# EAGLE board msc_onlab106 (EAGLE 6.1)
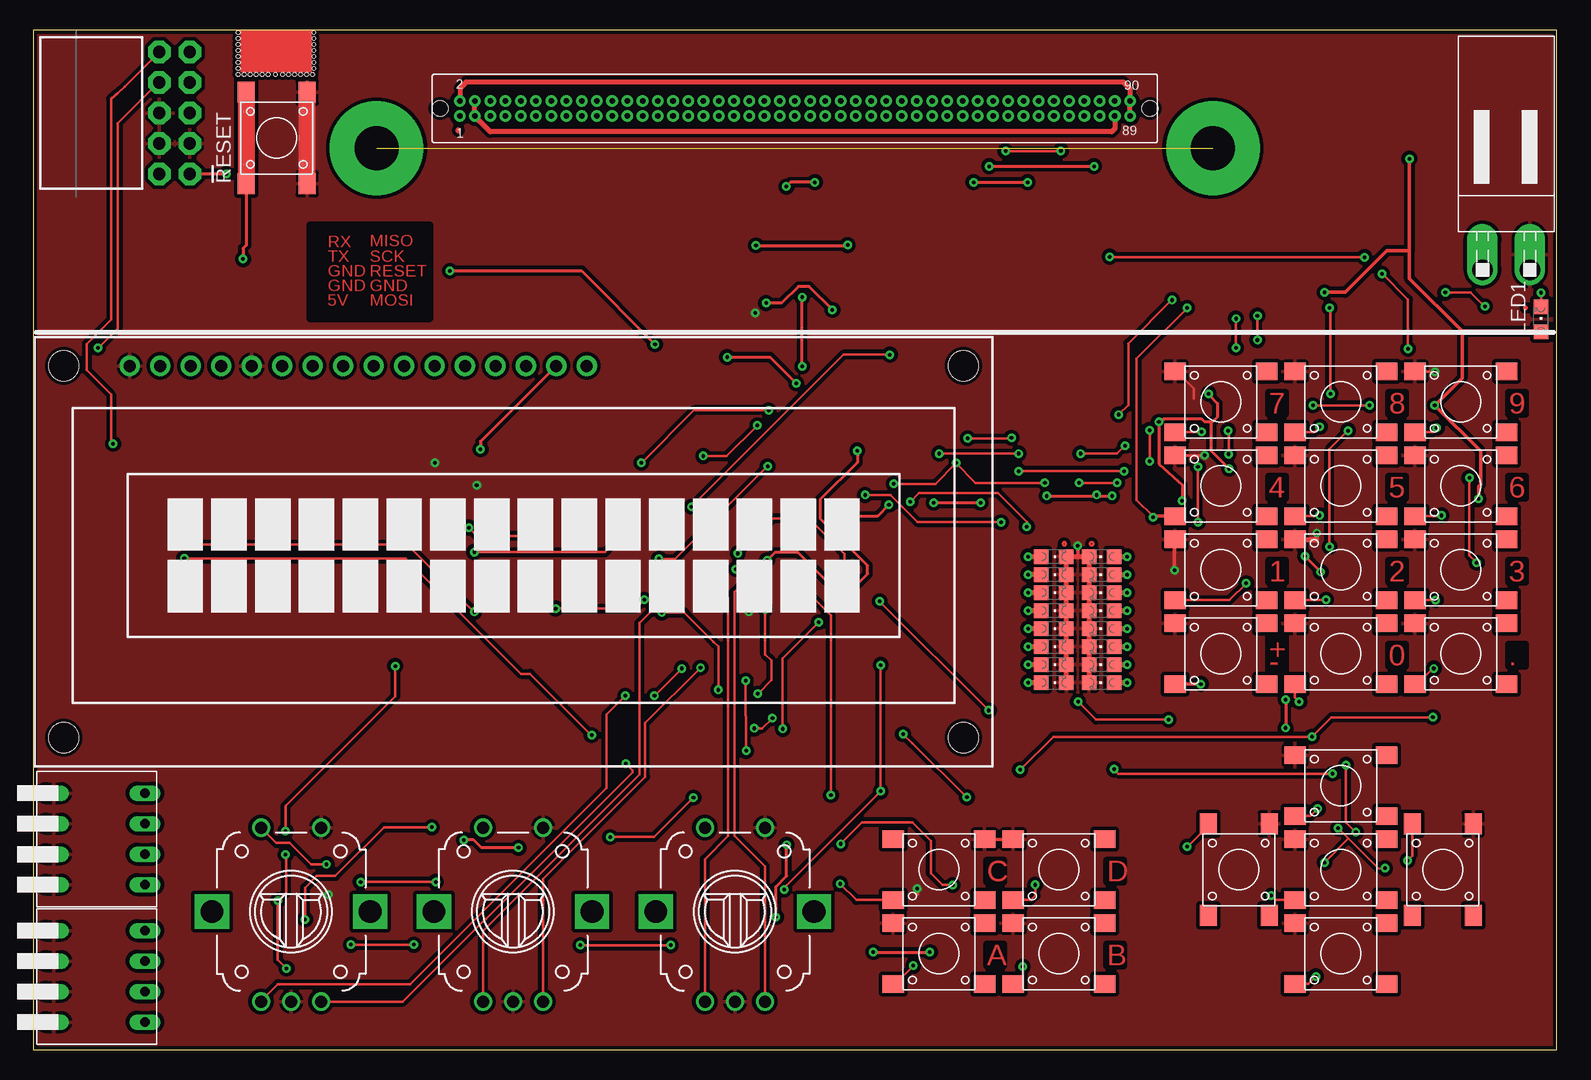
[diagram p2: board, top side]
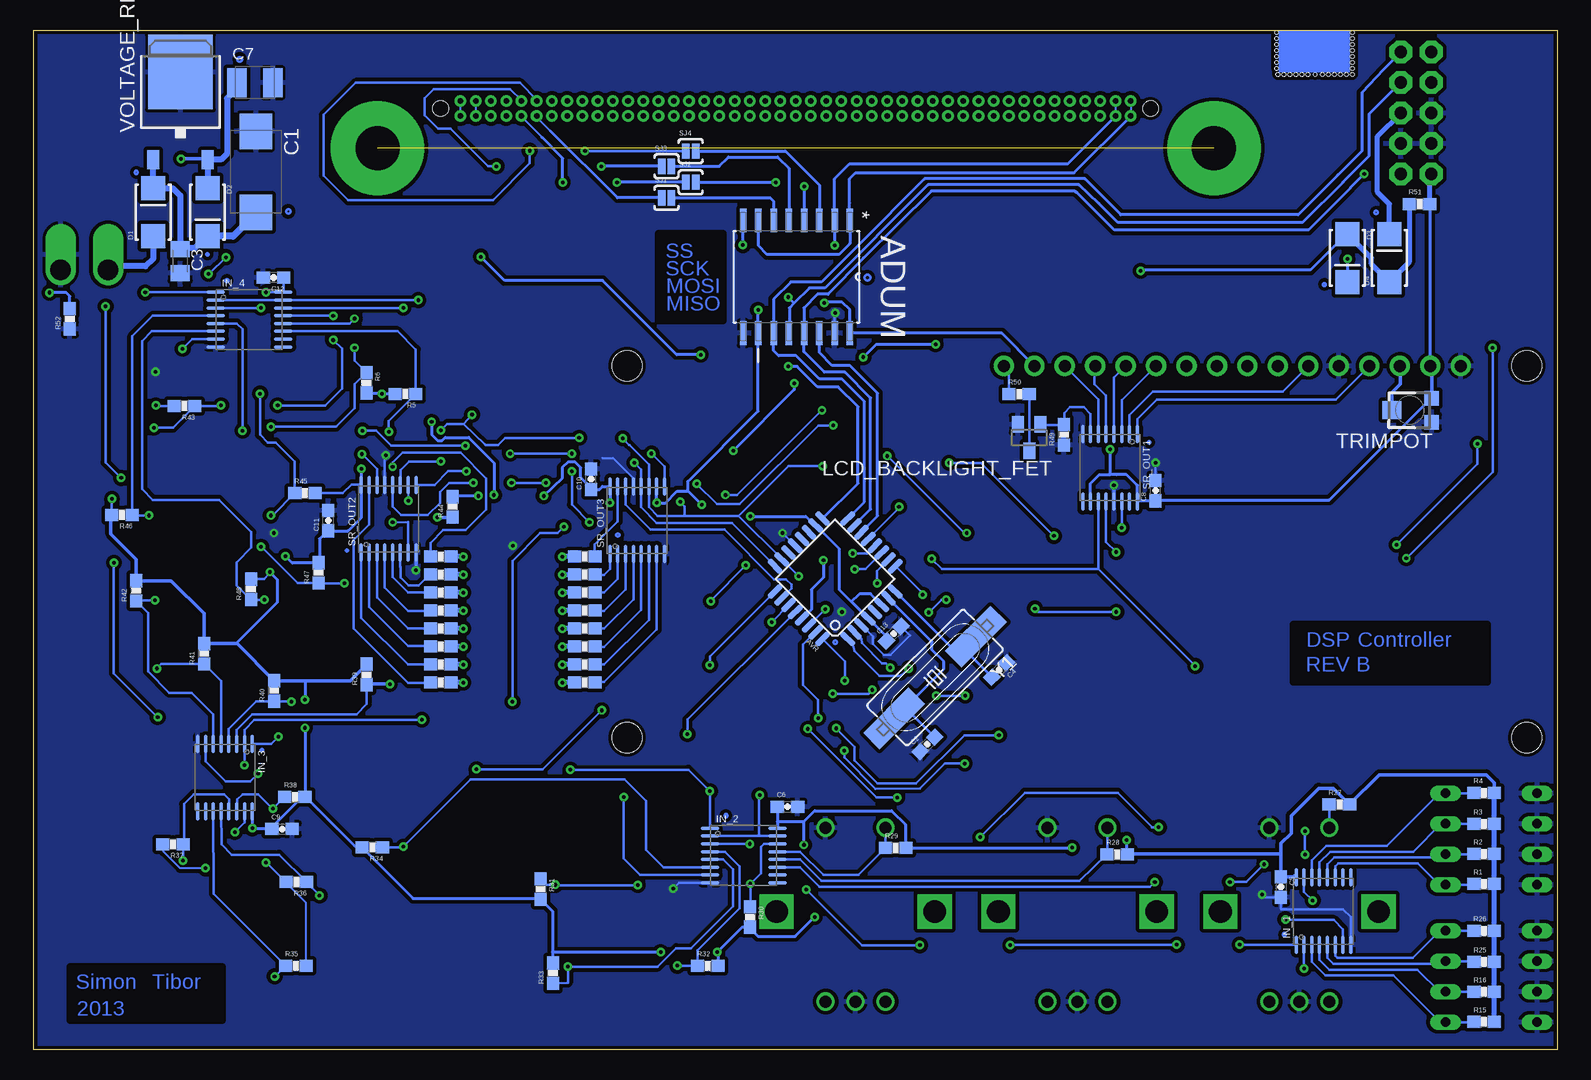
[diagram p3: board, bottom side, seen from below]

Size 127 x 85 mm. Coordinates in mm from the lower left corner, seen from the top.
Outline: 0,0 127,0 127,85 0,85 0,0
Copper layers (1*16): Top 0.035mm / dielectric 1.5mm / Bottom 0.035mm
Design rules: minimum track width 7mil, minimum drill 0.3mm, track to track 8mil, track to pad 8mil, pad to pad 7mil, via to via 7mil, smd to smd 7mil, copper to edge 10mil, drill to drill 7mil, minimum pad ring 10mil, minimum via ring 8mil, stop-mask expansion 2mil, vias tented up to drill 30mil, thermal gap 10mil
Holes 0.3 mm at 17.1,84.8 17.1,84.3 17.1,83.8 17.1,83.3 17.1,82.8 17.1,82.3 17.1,81.8 17.1,81.3 17.6,81.3 18.1,81.3 18.6,81.3 19.1,81.3 19.6,81.3 20.2,81.3 20.8,81.3 21.3,81.3 21.8,81.3 22.3,81.3 22.8,81.3 23.3,81.3 23.4,81.8 23.4,82.3 23.4,82.8 23.4,83.3 23.4,83.8 23.4,84.3 23.4,84.8
tRestrict: area 23.1,60.9 to 33.1,68.7
bRestrict: area 5.8,30.6 to 22,35.4; area 111.3,2.4 to 124,6.9; area 69.5,60.8 to 74.9,68

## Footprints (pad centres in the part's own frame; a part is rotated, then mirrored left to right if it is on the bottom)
SMD = smd 1.778 x 1.422: P$1 3.81,-2.54; P$2 -3.81,-2.54; P$3 3.81,2.54; P$4 -3.81,2.54
SOIC127P1032X265-16N = smd 1.981 x 0.533: 1 -4.699,4.445; 2 -4.699,3.175; 3 -4.699,1.905; 4 -4.699,0.635; 5 -4.699,-0.635; 6 -4.699,-1.905; 7 -4.699,-3.175; 8 -4.699,-4.445; 9 4.699,-4.445; 10 4.699,-3.175; 11 4.699,-1.905; 12 4.699,-0.635; 13 4.699,0.635; 14 4.699,1.905; 15 4.699,3.175; 16 4.699,4.445
TQFP32-08 = smd 1.524 x 0.559: 1 -4.293,2.8; 2 -4.293,2; 3 -4.293,1.2; 4 -4.293,0.4; 5 -4.293,-0.4; 6 -4.293,-1.2; 7 -4.293,-2; 8 -4.293,-2.8; 17 4.293,-2.8; 18 4.293,-2; 19 4.293,-1.2; 20 4.293,-0.4; 21 4.293,0.4; 22 4.293,1.2; 23 4.293,2; 24 4.293,2.8 | smd 0.559 x 1.524: 9 -2.8,-4.293; 10 -2,-4.293; 11 -1.2,-4.293; 12 -0.4,-4.293; 13 0.4,-4.293; 14 1.2,-4.293; 15 2,-4.293; 16 2.8,-4.293; 25 2.8,4.293; 26 2,4.293; 27 1.2,4.293; 28 0.4,4.293; 29 -0.4,4.293; 30 -1.2,4.293; 31 -2,4.293; 32 -2.8,4.293
D/7343-31W = smd 2.95 x 2.7: + 3.375,0; - -3.375,0
0603-CAP = smd 1.1 x 1: 1 -0.85,0; 2 0.85,0
C0805K = smd 1.3 x 1.6: 1 -1,0; 2 1,0
SMC_B = smd 1.6 x 2.4: + -1.5,0; - 1.5,0
SAMTEC-TFC = drill 0.46 pad 0.9: 1 27.94,0.635; 2 27.94,-0.635; 3 26.67,0.635; 4 26.67,-0.635; 5 25.4,0.635; 6 25.4,-0.635; 7 24.13,0.635; 8 24.13,-0.635; 9 22.86,0.635; 10 22.86,-0.635; 11 21.59,0.635; 12 21.59,-0.635; 13 20.32,0.635; 14 20.32,-0.635; 15 19.05,0.635; 16 19.05,-0.635; 17 17.78,0.635; 18 17.78,-0.635; 19 16.51,0.635; 20 16.51,-0.635; 21 15.24,0.635; 22 15.24,-0.635; 23 13.97,0.635; 24 13.97,-0.635; 25 12.7,0.635; 26 12.7,-0.635; 27 11.43,0.635; 28 11.43,-0.635; 29 10.16,0.635; 30 10.16,-0.635; 31 8.89,0.635; 32 8.89,-0.635; 33 7.62,0.635; 34 7.62,-0.635; 35 6.35,0.635; 36 6.35,-0.635; 37 5.08,0.635; 38 5.08,-0.635; 39 3.81,0.635; 40 3.81,-0.635; 41 2.54,0.635; 42 2.54,-0.635; 43 1.27,0.635; 44 1.27,-0.635; 45 0,0.635; 46 0,-0.635; 47 -1.27,0.635; 48 -1.27,-0.635; 49 -2.54,0.635; 50 -2.54,-0.635; 51 -3.81,0.635; 52 -3.81,-0.635; 53 -5.08,0.635; 54 -5.08,-0.635; 55 -6.35,0.635; 56 -6.35,-0.635; 57 -7.62,0.635; 58 -7.62,-0.635; 59 -8.89,0.635; 60 -8.89,-0.635; 61 -10.16,0.635; 62 -10.16,-0.635; 63 -11.43,0.635; 64 -11.43,-0.635; 65 -12.7,0.635; 66 -12.7,-0.635; 67 -13.97,0.635; 68 -13.97,-0.635; 69 -15.24,0.635; 70 -15.24,-0.635; 71 -16.51,0.635; 72 -16.51,-0.635; 73 -17.78,0.635; 74 -17.78,-0.635; 75 -19.05,0.635; 76 -19.05,-0.635; 77 -20.32,0.635; 78 -20.32,-0.635; 79 -21.59,0.635; 80 -21.59,-0.635; 81 -22.86,0.635; 82 -22.86,-0.635; 83 -24.13,0.635; 84 -24.13,-0.635; 85 -25.4,0.635; 86 -25.4,-0.635; 87 -26.67,0.635; 88 -26.67,-0.635; 89 -27.94,0.635; 90 -27.94,-0.635 | hole 1.3: -29.6,0; 29.587,0
SMA-DIODE_ALT = smd 2 x 2: A -2,0; C 2,0
DIP04PIANO = drill 0.8 long: 11 -3.81,-2.69; 12 -3.81,4.93; 21 -1.27,-2.69; 22 -1.27,4.93; 31 1.27,-2.69; 32 1.27,4.93; 41 3.81,-2.69; 42 3.81,4.93
PEC12_INCREMENTAL_ENCODER = drill 1: A -2.5,-7.5; B 2.5,-7.5; C 0,-7.5; P1 -2.5,7; P2 2.5,7 | drill 1.9 square: GND@1 -6.6,0; GND@2 6.6,0
TI_PW = smd 0.3 x 1.55: 1 -2.275,-2.8; 2 -1.625,-2.8; 3 -0.975,-2.8; 4 -0.325,-2.8; 5 0.325,-2.8; 6 0.975,-2.8; 7 1.625,-2.8; 8 2.275,-2.8; 9 2.275,2.825; 10 1.625,2.825; 11 0.975,2.825; 12 0.325,2.825; 13 -0.325,2.825; 14 -0.975,2.825; 15 -1.625,2.825; 16 -2.275,2.825
TUXGR_16X2_R2 = drill 1 pad 1.676: 1 -32,15.5; 2 -29.46,15.5; 3 -26.92,15.5; 4 -24.38,15.5; 5 -21.84,15.5; 6 -19.3,15.5; 7 -16.76,15.5; 8 -14.22,15.5; 9 -11.68,15.5; 10 -9.14,15.5; 11 -6.6,15.5; 12 -4.06,15.5; 13 -1.52,15.5; 14 1.02,15.5; 15 3.56,15.5; 16 6.1,15.5 | hole 2.5: -37.5,-15.5; 37.5,-15.5; -37.5,15.5; 37.5,15.5
SOT23 = smd 1 x 1.4: 1 -0.95,-1.1; 2 0.95,-1.1; 3 0,1.1
CHIPLED_0805 = smd 1.2 x 1.2: A 0,-1.05; C 0,1.05
NSL39_2_CONNECTOR = drill 1.7 offset: P$1 0,1.98; P$2 0,-1.98
2X5-RAF = drill 1.016 pad 1.88 octagon: 1 -1.27,5.08; 2 1.27,5.08; 3 -1.27,2.54; 4 1.27,2.54; 5 -1.27,0; 6 1.27,0; 7 -1.27,-2.54; 8 1.27,-2.54; 9 -1.27,-5.08; 10 1.27,-5.08
0603-RES = smd 1.1 x 1: 1 -0.85,0; 2 0.85,0
SJ_2S-NOTRACE = smd 0.635 x 1.27: 1 -0.401,0; 2 0.413,0
TC33X = smd 1.2 x 1.2: 1 -1,-1.825; 3 1,-1.825 | smd 1.5 x 1.6: 2 0,1.5
TO252 = smd 1 x 1.6: 1 -2.28,-4.8; 2 2.28,-4.8 | smd 5.4 x 6.2: 3 0,2.5
HC49UP = smd 5.334 x 1.93: 1 -4.826,0; 2 4.826,0

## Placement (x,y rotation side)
A1  TACTM-67N  [SMD]  109,22 0 top
A2  TACTM-67N  [SMD]  100.5,15 270 top
A3  TACTM-67N  [SMD]  109,15 0 top
A4  TACTM-67N  [SMD]  117.5,15 270 top
A5  TACTM-67N  [SMD]  109,8 0 top
ADUM  ADUM1401BRWZ  [SOIC127P1032X265-16N]  63.43,64.42 270 bottom
AVR  ATMEGA168  [TQFP32-08]  60.21,39.24 135 bottom
C1  47u  [D/7343-31W]  108.49,73.18 270 bottom
C2  22p  [0603-CAP]  52.51,25.44 45 bottom
C3  100n  [C0805K]  114.8,65.73 270 bottom
C4  22p  [0603-CAP]  46.54,31.65 225 bottom
C5  1u  [0603-CAP]  23.05,13.55 270 bottom
C6  1u  [0603-CAP]  64.18,20.24 0 bottom
C7  22u  [SMC_B]  108.57,80.61 0 bottom
C8  1u  [0603-CAP]  33.5,46.6 90 bottom
C9  1u  [0603-CAP]  106.31,18.38 0 bottom
C10  1u  [0603-CAP]  80.55,47.55 90 bottom
C11  1u  [0603-CAP]  102.45,44.1 90 bottom
C12  1u  [0603-CAP]  107.02,64.35 180 bottom
C13  1u  [0603-CAP]  55.33,34.67 45 bottom
CONNECTOR  SAMTEC_TFC  [SAMTEC-TFC]  63.5,78.46 180 top
D1  TACTM-67N  [SMA-DIODE_ALT]  117.05,69.81 90 bottom
D2  TACTM-67N  [SMA-DIODE_ALT]  112.53,69.81 270 bottom
D3  TACTM-67N  [SMA-DIODE_ALT]  17.5,66 270 bottom
D4  TACTM-67N  [SMA-DIODE_ALT]  14,66 90 bottom
DIP1  DIP04PIANO  [DIP04PIANO]  4.39,17.55 270 top
DIP2  DIP04PIANO  [DIP04PIANO]  4.39,6.09 270 top
E1  ENCODER_SW1-PEC12  [PEC12_INCREMENTAL_ENCODER]  21.5,11.5 0 top
E2  ENCODER_SW1-PEC12  [PEC12_INCREMENTAL_ENCODER]  40,11.5 0 top
E3  ENCODER_SW1-PEC12  [PEC12_INCREMENTAL_ENCODER]  58.5,11.5 0 top
F1  TACTM-67N  [SMD]  75.5,15 0 top
F2  TACTM-67N  [SMD]  85.5,15 0 top
F3  TACTM-67N  [SMD]  75.5,8 0 top
F4  TACTM-67N  [SMD]  85.5,8 0 top
IN_1  74HC165  [TI_PW]  19.5,11.54 0 bottom
IN_2  74HC165  [TI_PW]  67.85,16.17 270 bottom
IN_3  74HC165  [TI_PW]  111.07,22.67 180 bottom
IN_4  74HC165  [TI_PW]  109.04,60.86 270 bottom
LCD  RC-1602-BB  [TUXGR_16X2_R2]  40.05,41.5 0 top
LCD_BACKLIGHT_FET  BSS 138  [SOT23]  44.03,51.02 180 bottom
LED1  [CHIPLED_0805]  125.68,60.87 0 top
LED17  OF-SMD 2012 R/Y/G  [CHIPLED_0805]  89.08,30.59 90 top
LED18  OF-SMD 2012 R/Y/G  [CHIPLED_0805]  89.08,32.09 90 top
LED19  OF-SMD 2012 R/Y/G  [CHIPLED_0805]  89.08,33.59 90 top
LED20  OF-SMD 2012 R/Y/G  [CHIPLED_0805]  89.08,35.09 90 top
LED21  OF-SMD 2012 R/Y/G  [CHIPLED_0805]  89.08,36.59 90 top
LED22  OF-SMD 2012 R/Y/G  [CHIPLED_0805]  89.08,38.09 90 top
LED23  OF-SMD 2012 R/Y/G  [CHIPLED_0805]  89.08,39.59 90 top
LED24  OF-SMD 2012 R/Y/G  [CHIPLED_0805]  89.08,41.09 90 top
LED25  OF-SMD 2012 R/Y/G  [CHIPLED_0805]  85.08,41.09 270 top
LED26  OF-SMD 2012 R/Y/G  [CHIPLED_0805]  85.08,39.59 270 top
LED27  OF-SMD 2012 R/Y/G  [CHIPLED_0805]  85.08,38.09 270 top
LED28  OF-SMD 2012 R/Y/G  [CHIPLED_0805]  85.08,36.59 270 top
LED29  OF-SMD 2012 R/Y/G  [CHIPLED_0805]  85.08,35.09 270 top
LED30  OF-SMD 2012 R/Y/G  [CHIPLED_0805]  85.08,33.59 270 top
LED31  OF-SMD 2012 R/Y/G  [CHIPLED_0805]  85.08,32.09 270 top
LED32  OF-SMD 2012 R/Y/G  [CHIPLED_0805]  85.08,30.59 270 top
N1  TACTM-67N  [SMD]  99,54 0 top
N2  TACTM-67N  [SMD]  109,54 0 top
N3  TACTM-67N  [SMD]  119,54 0 top
N4  TACTM-67N  [SMD]  99,47 0 top
N5  TACTM-67N  [SMD]  109,47 0 top
N6  TACTM-67N  [SMD]  119,47 0 top
N7  TACTM-67N  [SMD]  99,40 0 top
N8  TACTM-67N  [SMD]  109,40 0 top
N9  TACTM-67N  [SMD]  119,40 0 top
N10  TACTM-67N  [SMD]  99,33 0 top
N11  TACTM-67N  [SMD]  109,33 0 top
N12  TACTM-67N  [SMD]  119,33 0 top
POWER_CONNECTOR  NSL39_2_CONNECTOR  [NSL39_2_CONNECTOR]  122.79,64.99 270 top
PROGRAMMING_CONNECTOR  M05X2RAF  [2X5-RAF]  11.78,78.08 180 top
R1  10k  [0603-RES]  6.1,13.8 0 bottom
R2  10k  [0603-RES]  6.1,16.3 0 bottom
R3  10k  [0603-RES]  6.1,18.8 0 bottom
R4  10k  [0603-RES]  6.1,21.4 0 bottom
R5  10k  [0603-RES]  96.03,54.66 180 bottom
R6  10k  [0603-RES]  99.28,55.6 270 bottom
R7  1k  [0603-RES]  93.08,30.59 0 bottom
R8  1k  [0603-RES]  93.08,32.09 0 bottom
R9  1k  [0603-RES]  93.08,33.59 0 bottom
R10  1k  [0603-RES]  93.08,35.09 0 bottom
R11  1k  [0603-RES]  93.08,36.59 0 bottom
R12  1k  [0603-RES]  93.08,38.09 0 bottom
R13  1k  [0603-RES]  93.08,39.59 0 bottom
R14  1k  [0603-RES]  93.08,41.09 0 bottom
R15  10k  [0603-RES]  6.1,2.3 0 bottom
R16  10k  [0603-RES]  6.1,4.8 0 bottom
R17  1k  [0603-RES]  81.08,41.09 180 bottom
R18  1k  [0603-RES]  81.08,39.59 180 bottom
R19  1k  [0603-RES]  81.08,38.09 180 bottom
R20  1k  [0603-RES]  81.08,36.59 180 bottom
R21  1k  [0603-RES]  81.08,35.09 180 bottom
R22  1k  [0603-RES]  81.08,33.59 180 bottom
R23  1k  [0603-RES]  81.08,32.09 180 bottom
R24  1k  [0603-RES]  81.08,30.59 180 bottom
R25  10k  [0603-RES]  6.1,7.3 0 bottom
R26  10k  [0603-RES]  6.1,9.9 0 bottom
R27  10k  [0603-RES]  18.18,20.43 0 bottom
R28  10k  [0603-RES]  36.69,16.27 0 bottom
R29  10k  [0603-RES]  55.15,16.82 0 bottom
R30  10k  [0603-RES]  67.31,11.06 270 bottom
R31  10k  [0603-RES]  84.76,13.37 270 bottom
R32  10k  [0603-RES]  70.82,6.98 0 bottom
R33  10k  [0603-RES]  83.71,6.36 90 bottom
R34  10k  [0603-RES]  98.79,16.86 180 bottom
R35  10k  [0603-RES]  105.16,6.98 0 bottom
R36  10k  [0603-RES]  105.13,13.96 180 bottom
R37  10k  [0603-RES]  115.41,17.12 180 bottom
R38  10k  [0603-RES]  105.25,21.06 0 bottom
R39  10k  [0603-RES]  99.26,31.27 90 bottom
R40  10k  [0603-RES]  106.98,29.9 90 bottom
R41  10k  [0603-RES]  112.81,32.99 90 bottom
R42  10k  [0603-RES]  118.47,38.24 90 bottom
R43  10k  [0603-RES]  114.45,53.64 180 bottom
R44  10k  [0603-RES]  92.08,45.24 90 bottom
R45  10k  [0603-RES]  104.39,46.39 0 bottom
R46  10k  [0603-RES]  119.66,44.58 180 bottom
R47  10k  [0603-RES]  103.26,39.74 90 bottom
R48  10k  [0603-RES]  108.91,38.36 90 bottom
R49  10k  [0603-RES]  41.14,51.24 90 bottom
R50  20  [0603-RES]  44.88,54.64 0 bottom
R51  10k  [0603-RES]  11.5,70.5 0 bottom
R52  550  [0603-RES]  124,60.93 90 bottom
RESET  NSG 39-2  [SMD]  20.3,76 90 top
SJ1  SOLDERJUMPERNC2  [SJ_2S-NOTRACE]  74.26,71 0 bottom
SJ2  SOLDERJUMPERNC2  [SJ_2S-NOTRACE]  72.25,72.3 0 bottom
SJ3  SOLDERJUMPERNC2  [SJ_2S-NOTRACE]  74.26,73.64 0 bottom
SJ4  SOLDERJUMPERNC2  [SJ_2S-NOTRACE]  72.25,74.9 0 bottom
SR_OUT1  74HC595  [TI_PW]  37.29,48.51 180 bottom
SR_OUT2  74HC595  [TI_PW]  97.42,44.25 0 bottom
SR_OUT3  74HC595  [TI_PW]  76.7,44.12 0 bottom
TRIMPOT  10k  [TC33X]  12.3,53.3 90 bottom
VOLTAGE_REGULATOR  7805DT  [TO252]  114.78,78.99 0 bottom
Y1  16MHz  [HC49UP]  51.88,31.01 225 bottom

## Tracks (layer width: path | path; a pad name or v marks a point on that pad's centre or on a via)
3V3
  Top 0.254: 35.55,79.1 CONNECTOR.2
  Top 0.406: CONNECTOR.89 91.44,79.06 91.45,79.06 91.45,80.08 90.88,80.65 36.08,80.65 35.59,80.16 35.59,79.14 35.55,79.1
  Bottom 0.178: CONNECTOR.90 CONNECTOR.89 | CONNECTOR.2 CONNECTOR.1
  Bottom 0.254: CONNECTOR.1 40.28,73.1 58.5,73.1 59,72.6 59,70.58 ADUM.1 58.99,67.2 59.9,66.29 65.88,66.29 66.59,67 66.59,69.1 ADUM.7
3V3_GND  (via drill 0.3)
  Top 0.254: 36.81,79.1 36.82,79.1 CONNECTOR.4 | v60.26,67.04 67.86,67.04 v67.89,67.07
  Top 0.406: CONNECTOR.87 90.17,76.77 89.9,76.5 38.11,76.5 36.81,77.8 36.81,79.1
  Bottom 0.178: CONNECTOR.88 CONNECTOR.87 | CONNECTOR.4 CONNECTOR.3
  Bottom 0.254: CONNECTOR.3 40.8,73.85 59,73.85 60.26,72.59 ADUM.2 v60.26,67.04 | v67.89,67.07 67.89,69.1 ADUM.8
5V  (via drill 0.3)
  Top 0.178: 43.55,56.96 LCD.15 | v112.69,15.11 112.12,15.11 109.65,17.59 | v108.79,18.44 109.65,17.59 | 109.65,17.59 v107.66,15.6 | 98.31,52.33 98.23,52.33 | 97.99,54.6 v97.99,54.68 | v88.64,46.23 88.64,46.15 | v93.84,52.33 93.92,52.24 93.84,52.24
  Top 0.203: v97.99,54.68 97.83,54.68 | v116.84,53.71 116.76,53.71 116.67,53.62 | v120.49,45.91 120.49,45.74 | v107.66,63.13 107.58,63.13 | v95.79,45.74 95.79,45.91
  Top 0.254: v61.1,62.24 62.4,62.24 63.78,63.62 64.67,63.62 v66.62,61.67 | v37.29,50.05 37.29,50.7 43.55,56.96 | v70.04,8.12 v74.75,8.12 | v62.81,17.06 62.81,14.46 61.91,13.57 v61.91,11.05 | v84.5,46.15 88.64,46.15 v89.94,46.15 | v78.97,45.58 v75.08,45.58 | v67.28,44.44 70.36,44.44 v71.34,45.42 | v95.79,45.74 95.79,47.04 93.84,48.83 93.84,52.24 94.25,52.57 97.42,52.57 97.66,52.33 98.23,52.33 98.23,49.89 v99.69,48.42 | 98.31,52.33 98.72,52.73 98.72,53.87 97.99,54.6 | v106.03,41.11 v107.33,39.81 | v104.41,29.17 v104.41,26.81 | v35.91,17.47 36.73,17.47 37.38,16.82 v40.46,16.82
  Top 0.305: v114.72,74.26 114.72,66.62 | 119.11,59.88 114.72,64.27 114.72,66.62 | 119.11,59.88 125.61,59.88 LED1.A | LED1.A | LED1.A 125.69,59.8 | 114.72,66.62 112.86,66.62 109.36,63.13 v107.66,63.13 | 119.11,59.88 119.11,55.98 v116.84,53.71 120.66,49.89 120.66,47.12 120.49,46.96 v120.49,45.91
  Bottom 0.178: 66.62,59.88 66.54,59.8 ADUM.10 66.62,59.64 | 58.99,59.8 ADUM.16 58.91,59.72 | 10.64,57.12 LCD.2 | 10.64,70.36 R51.2 | 38.92,46.31 SR_OUT1.10 | 36.64,47.94 36.73,47.94 | 10.89,53.95 10.56,54.19 TRIMPOT.3 | 33.48,45.83 C8.1 | 43.63,57.04 LCD.15 | 54.36,16.82 R29.2 54.27,16.82 | 83.77,7.23 R33.2 | 84.74,12.51 R31.2 84.83,12.59 | 69.96,6.99 R32.2 | v70.04,8.12 69.96,8.12 | 67.44,10.56 R30.2 | 92.06,46.15 R44.2 | 80.52,46.8 C10.1 | 61.91,43.71 AVR.18 | 74.99,45.58 v75.08,45.58 | 100.18,16.9 99.69,16.9 R34.2 99.61,16.82 | 104.33,21.04 R38.2 | R35.2 104.33,6.99 104.33,12.27 105.95,13.89 R36.2 106.03,13.97 v107.66,15.6 | 107.58,18.44 107.17,18.61 C9.1 107.09,18.61 | 108.79,19.82 IN_3.16 | v112.69,15.11 114.81,15.11 116.19,16.49 116.19,17.06 R37.2 | 104.65,21.04 104.49,21.04 R38.2 | v95.79,45.74 95.79,47.04 SR_OUT2.10 | 103.19,40.62 R47.2 103.27,40.54 | 102.54,43.23 C11.1 | 108.88,39.24 R48.2 | 99.69,47.12 SR_OUT2.16 | 110.01,33.96 110.07,33.84 | 104.41,21.12 R38.2
  Bottom 0.203: 97.96,54.66 v97.99,54.68 | v97.99,54.69 v97.99,54.68 | R43.2 116.78,53.64 v116.84,53.71 | 98.06,54.75 v97.99,54.68 | R46.2 120.51,45.89 v120.49,45.91 | IN_4.16 106.28,63.13 | 106.28,63.13 v107.66,63.13 | 21.9,14.4 21.8,14.3 21.8,14.35 21.79,14.35 IN_1.16 | C13.1 55.93,34.43 | 57.45,35.95 57.35,35.85 57.38,35.85 AVR.4 | 34.9,45.75 35,45.65 35,45.7 SR_OUT1.16 | SR_OUT3.16 | SR_OUT2.16 99.69,47.04 99.78,47.12 100.51,47.12 101.24,46.39 R45.2 | SR_OUT2.16 99.7,47.12 99.69,47.12 SR_OUT2.16 | 65.03,18.46 IN_2.16 | C12.1 106.17,63.24 106.28,63.13 | 35.9,16.74 R28.2 | 61.02,62.32 v61.1,62.24 | 108.88,39.24 107.82,39.24 107.33,39.73 v107.33,39.81
  Bottom 0.254: R5.2 97.96,54.66 | R6.2 98.06,54.75 | AVR.18 61.81,43.69 59.88,41.76 59.88,38.35 AVR.4 57.45,35.96 58.83,37.33 58.17,37.98 57.24,37.98 AVR.6 | 55.93,34.43 57.35,35.85 | C8.1 34.9,45.75 | C10.1 79.85,46.7 79.6,46.95 SR_OUT3.16 | C11.1 100.81,43.25 99.69,44.36 99.69,47.04 | C6.1 65.03,19.01 | 65.03,19.01 65.03,18.46 | 66.62,59.88 v66.62,61.67 | 10.64,70.36 10.64,57.12 | 37.29,47.94 36.73,47.94 35.91,47.94 35,47.02 35,45.7 | v37.29,50.05 37.29,47.94 | 10.89,53.95 19.01,45.83 33.48,45.83 | 58.91,59.72 46.31,59.72 43.63,57.04 | 54.36,16.82 54.36,18.77 55.49,19.91 61.91,19.91 62.81,19.01 | 65.03,19.01 62.81,19.01 | 83.77,8.12 83.77,11.54 84.74,12.51 | 83.77,8.12 83.77,7.23 | 69.96,8.12 69.96,6.99 | v74.75,8.12 83.77,8.12 | v62.81,17.06 62.81,19.01 | v61.91,11.05 63.54,9.43 66.62,9.43 67.36,10.16 R30.2 | v89.94,46.15 92.06,46.15 | v84.5,46.15 82.96,47.61 82.96,48.51 82.47,48.99 81.9,48.99 81.41,48.51 81.41,47.69 80.52,46.8 | v75.08,45.58 SR_OUT3.10 | SR_OUT3.16 v78.97,45.58 | 61.91,43.71 62.64,44.44 v67.28,44.44 | 72.47,46.56 v71.34,45.42 | 72.47,46.56 73.37,46.56 74.34,45.58 74.99,45.58 | 104.33,21.04 100.18,16.9 | 107.09,18.61 104.65,21.04 | 103.19,40.62 103.19,42.58 102.54,43.23 | 99.69,47.12 v99.69,48.42 | 110.01,33.96 106.68,37.29 106.68,39.16 v107.33,39.81 | v104.41,26.81 104.41,21.12 | 104.41,30.75 v104.41,29.17 | v88.64,46.23 88.64,48.91 90.76,51.02 92.71,51.02 92.95,50.78 93.36,50.78 93.84,51.27 v93.84,52.33 | 84.83,12.59 95.39,12.59 99.61,16.82 | 54.27,16.82 v40.46,16.82 | 66.62,59.64 66.62,53.22 72.47,47.37 72.47,46.56 | 58.99,59.8 58.99,61.67 59.64,62.32 61.02,62.32 | 103.27,40.54 105.46,40.54 v106.03,41.11
  Bottom 0.254: 107.58,18.44 v108.79,18.44 108.79,19.82 | 35.9,16.74 35.9,17.46 v35.91,17.47 | R30.2 67.96,10.21 v70.04,8.12 | R30.2 67.28,10.24 | 38.92,46.31 38.92,47.21 38.19,47.94 37.29,47.94
  Bottom 0.305: TRIMPOT.3 10.47,56.88 LCD.2 | D2.A 112.53,74.26 v114.72,74.26 | R46.2 120.58,44.51 120.58,42.98 118.47,40.88 R42.2 115.54,39.08 112.81,36.36 R41.2 110.07,33.84 R40.2 104.41,30.75 100.62,30.75 R39.2 | R4.2 5.25,22.23 5.93,22.91 14.84,22.91 R27.2 18.68,21.77 19.91,21.77 22.18,19.5 22.18,18.04 23.05,17.17 23.05,16.31 | 21.88,14.4 C5.1 23.05,16.31 | 21.88,14.4 21.86,14.38 | 21.88,14.4 21.94,14.46 21.88,14.46 IN_1.16 | 23.05,16.31 35.47,16.31 R28.2
  Bottom 0.406: R51.2 10.65,72.86 PROGRAMMING_CONNECTOR.2 | R15.2 R16.2 R25.2 R26.2 R1.2 R2.2 R3.2 R4.2
  Bottom 0.508: D2.A 112.5,71.83 VOLTAGE_REGULATOR.2 111.4,74.2 110.9,74.7 110.9,79.3 110.07,80.13 C7.+
CLK3
  Bottom 0.254: SJ3.2 69.88,73.64 69.09,74.42 65,74.42 64.06,73.47 64.06,69.18 64.09,69.15 64.09,69.14 ADUM.5
GND  (via drill 0.3)
  Top 0.203: N4.P$4 96.46,49.54 v97.65,49.54 | 106.83,49.54 106.88,49.5 | N3.P$4 116.83,56.54 | N1.P$4 95.32,56.54 96.77,55.09 96.77,54.27 | v24.62,12.92 24.7,12.92 24.78,12.84 | v33.48,48.91 33.48,48.99 | v60.21,61.42 60.21,61.1 | v73.69,13.41 73.69,13 73.78,12.92 | v64.59,43.06 64.51,43.14
  Top 0.254: F1.P$3 81.56,17.54 81.6,17.5 81.7,17.5 | 81.8,17.5 81.7,17.5 | 81.7,17.5 F2.P$4
  Top 0.305: LED25.C 87.08,41.09 87.08,41.11 v87.08,42.01 | v95.14,39.98 95.14,42.49 95.22,42.58 | v36.97,47.04 36.97,46.8
  Top 0.406: LED17.C LED18.C LED19.C LED20.C LED21.C LED22.C LED23.C LED24.C LED25.C LED26.C LED27.C LED28.C LED29.C LED30.C LED31.C LED32.C | N8.P$4 107.01,42.54 v107.01,43.06
  Top 1.42: RESET.P$2 RESET.P$1
  Bottom 0.178: SR_OUT3.13 77.03,47.61 78.73,49.32 79.62,49.32 | 80.52,48.42 C10.2
  Bottom 0.203: SR_OUT2.13 97.75,49.44 v97.65,49.54 | AVR.3 57.95,35.36 57.04,34.45 57.04,33.8 56.14,32.91 55.58,32.91 53.95,34.53 53.98,34.53 C13.2 | 17.23,8.69 17.23,11.05 17.88,11.7 22.99,11.7 23.05,11.76 C5.2 24.4,12.7 v24.62,12.92 | C8.2 33.5,48.89 v33.48,48.91 | ADUM.15 60.26,61.21 v60.21,61.42 | IN_2.8 73.2,13.9 v73.69,13.41 | AVR.21 v64.59,43.06
  Bottom 0.305: SR_OUT2.8 v95.15,39.98 v95.14,39.98 | SR_OUT1.13 v36.97,47.04
  Bottom 0.406: v107.01,43.06 106.92,43.06 106.92,42.98
  other vias: 116.88,56.5 59.64,36.48
  pour Bottom (isolate 0.305): 0,85 127,85 127,0 0,0
  pour Top (isolate 0.305): 0,85 127,85 127,0 0,0 0,0.1
IN1A
  Bottom 0.203: IN_1.11 18.52,15.28 18.28,15.52 11.62,15.52 9.8,13.7 9.4,13.7 | 9.4,13.7 8.09,13.7 8.05,13.74 7.01,13.74 R1.1 | DIP1.42 9.36,13.74 9.4,13.7
IN1B
  Bottom 0.203: IN_1.12 19.18,15.44 18.61,16.01 9.99,16.01 9.7,16.3 9.3,16.3 | 9.3,16.3 8.07,16.3 8.05,16.28 6.97,16.28 R2.1 | DIP1.32 9.3,16.3
IN1C
  Bottom 0.203: IN_1.13 19.82,15.6 18.93,16.49 12.01,16.49 9.7,18.8 9.3,18.8 | 9.3,18.8 8.1,18.8 | 8.1,18.8 8.07,18.8 | 8.07,18.8 8.05,18.82 8.05,18.85 8.1,18.8 | 8.07,18.8 R3.1 | DIP1.22 9.3,18.8
IN1D
  Bottom 0.203: IN_1.14 20.48,15.76 19.26,16.98 14.22,16.98 9.84,21.36 | 9.84,21.36 9.8,21.4 8.09,21.4 8.05,21.36 6.99,21.36 R4.1 | DIP1.12 9.84,21.36
IN1E
  Bottom 0.203: IN_1.3 20.48,7.31 19.34,6.17 13.68,6.17 9.8,2.3 | 9.8,2.3 8.06,2.3 8.05,2.28 6.97,2.28 R15.1 | DIP2.42 9.78,2.28 9.8,2.3
IN1F
  Bottom 0.203: IN_1.4 19.82,7.47 19.01,6.66 11.66,6.66 9.82,4.82 | 9.82,4.82 9.8,4.8 8.07,4.8 8.05,4.82 6.97,4.82 R16.1 | DIP2.32 9.82,4.82
IN1G
  Bottom 0.203: IN_1.5 19.18,7.64 18.69,7.15 9.85,7.15 9.7,7.3 | 9.7,7.3 8.11,7.3 8.05,7.36 7.01,7.36 R25.1 | DIP2.22 9.64,7.36 9.7,7.3
IN1H
  Bottom 0.203: IN_1.6 18.52,7.8 18.36,7.64 12.06,7.64 9.8,9.9 9.4,9.9 | 9.4,9.9 8.05,9.9 8,9.9 R26.1 | DIP2.12 9.4,9.9
IN2A  (via drill 0.3)
  Top 0.203: v33.56,13.97 v27.3,13.97 | 19.02,18.52 E1.P1 20.27,17.23 21.37,17.23 23.16,15.44 v24.46,15.44
  Bottom 0.203: R27.1 19.02,18.52 E1.P1 | IN_2.11 63.14,15.2 61.51,13.57 33.96,13.57 v33.56,13.97 | v27.3,13.97 25.92,13.97 v24.46,15.44
IN2B
  Bottom 0.203: E2.P1 37.52,16.38 R28.1 39.84,14.06 61.34,14.06 63.14,15.85 IN_2.12
IN2C
  Bottom 0.203: E3.P1 56,16.84 55.98,16.82 R29.1 58.27,14.54 61.18,14.54 63.14,16.5 IN_2.13
IN2D  (via drill 0.3)
  Top 0.203: F1.P$2 68.63,12.46 v67.28,13.81
  Bottom 0.203: R30.1 67.28,12.51 v67.28,13.81 66.38,14.71 66.38,16.9 66.13,17.15 IN_2.14
IN2E  (via drill 0.3)
  Top 0.203: v67.31,17.14 69.1,18.93 73.29,18.93 74.83,17.39 74.83,14.71 75.81,13.73 76.62,13.73 v76.65,13.7 | F2.P$2 83.16,12.46 83.55,12.85 83.55,13.71 v83.53,13.73
  Bottom 0.203: v67.31,17.14 IN_2.3 | 84.83,14.22 84.34,13.73 v83.53,13.73 83.49,13.7 v76.65,13.7
  Bottom 0.254: 84.83,14.22 R31.1 | R31.1 84.72,14.22 84.7,14.2 84.74,14.2 R31.1
IN2F  (via drill 0.3)
  Top 0.203: F3.P$2 71.84,5.46 v73.37,6.99
  Bottom 0.203: v73.37,6.99 R32.1 | R32.1 | R32.1 71.67,8.28 68.17,11.78 68.17,15.28 69.39,16.49 IN_2.4
IN2G  (via drill 0.3)
  Top 0.203: F4.P$2 82.49,5.86 v82.49,6.91
  Bottom 0.203: R33.1 83.71,5.53 82.49,5.58 v82.49,6.91 74.99,6.91 73.45,8.45 72.23,8.45 68.74,11.94 68.74,15.03 69.55,15.84 IN_2.5
IN2H  (via drill 0.3)
  Top 0.203: 97.96,18.82 97.58,18.44 97.58,18.28 v96.2,16.9 | 97.99,18.77 97.99,18.85 97.96,18.82 | A2.P$2 97.96,18.82
  Bottom 0.203: R34.1 96.48,16.86 v96.2,16.9 90.59,22.51 77.76,22.51 75.97,20.72 75.97,16.66 74.51,15.2 IN_2.6
IN3C  (via drill 0.3)
  Top 0.203: A4.P$2 114.96,16.16 v114.56,15.76
  Bottom 0.203: v114.56,15.76 R37.1 114.48,17.2 114.48,20.48 113.67,21.29 111.15,21.29 110.71,20.84 IN_3.13
IN3D  (via drill 0.3)
  Top 0.203: A1.P$2 106.48,19.46 v107.09,20.07
  Bottom 0.203: R38.1 v107.09,20.07 108.31,21.29 109.61,21.29 110.06,20.84 IN_3.14
IN3E  (via drill 0.3)
  Top 0.305: N10.P$2 v97.34,30.46 v97.34,30.47
  Bottom 0.203: R39.1 99.26,28.79 100.1,27.95 108.79,27.95 110.09,26.65 IN_3.3 110.09,25.43
  Bottom 0.305: v97.34,30.47 99.26,30.47 R39.1
IN3F  (via drill 0.3)
  Top 0.203: N11.P$2 105.19,29.36 v105.54,29.01
  Bottom 0.203: v105.54,29.01 106.94,29.01 R40.1 107.03,29.01 108.47,29.01 110.74,26.73 IN_3.4
IN3G  (via drill 0.3)
  Top 0.203: v116.76,31.77 116.67,31.77 115.38,30.47 N12.P$2
  Bottom 0.203: IN_3.5 111.39,30.72 R41.1 116.39,32.14 v116.76,31.77
IN3H  (via drill 0.3)
  Top 0.203: N9.P$2 v116.92,37.46
  Bottom 0.203: v116.92,37.46 118.4,37.46 R42.1 118.38,37.3 118.38,37.29 117.49,36.4 117.49,31.52 115.7,29.74 113.83,29.74 112.04,27.95 IN_3.6
IN4A  (via drill 0.3)
  Top 0.203: N1.P$2 97.37,51.46 v97.42,51.51
  Bottom 0.203: IN_4.11 96.69,59.88 95.17,58.37 R5.1 97.42,52.41 v97.42,51.51
IN4B  (via drill 0.3)
  Top 0.203: N2.P$2 106.79,51.46 v107.25,51.92 | v100.26,60.94 v100.26,58.5
  Bottom 0.203: v107.25,51.92 101.81,51.92 100.26,53.46 100.26,55.47 R6.1 99.29,56.47 100.26,57.44 v100.26,58.5 | IN_4.12 100.67,60.53 v100.26,60.94
IN4C  (via drill 0.3)
  Top 0.203: N3.P$2 116.62,51.46 v117,51.84 | v102.05,59.15 v102.05,61.18 | v111.39,53.71 v106.68,53.71
  Bottom 0.203: v117,51.84 115.41,51.84 R43.1 111.46,53.64 v111.39,53.71 | v102.05,61.18 IN_4.13 | v102.05,59.15 101.32,58.42 101.32,55.09 102.7,53.71 v106.68,53.71
IN4D  (via drill 0.3)
  Top 0.203: v96.2,61.83 91.97,57.61 91.97,45.83 93.34,44.46 93.38,44.46
  Top 0.305: N4.P$2 93.38,44.46 v93.38,44.38
  Bottom 0.203: v96.2,61.83 IN_4.14
  Bottom 0.305: v93.38,44.38 92.08,44.38 R44.1
IN4E  (via drill 0.3)
  Top 0.203: N5.P$2 107.19,44.46 v107.25,44.52 | v108.14,54.68 108.14,61.75 v108.06,61.83
  Bottom 0.203: v107.25,44.52 107.11,44.52 R45.1 105.24,49.02 106.84,50.62 107.49,50.62 108.14,51.27 v108.14,54.68 | v108.06,61.83 IN_4.3
IN4F  (via drill 0.3)
  Top 0.203: N6.P$2 117.34,44.46 v117.41,44.52
  Bottom 0.203: v117.41,44.52 118.79,44.52 118.79,44.56 | 118.79,44.56 118.79,59.48 117.08,61.18 IN_4.4 111.8,61.18 | 118.79,44.56 R46.1
IN4G  (via drill 0.3)
  Top 0.203: N7.P$2 99.71,37.46 v101.12,38.88 | v108.06,41.92 108.06,50.05 v109.61,51.59
  Bottom 0.203: v101.12,38.88 103.25,38.88 R47.1 105.03,38.89 v108.06,41.92 | v109.61,51.59 109.61,60.04 110.09,60.53 IN_4.5
IN4H  (via drill 0.3)
  Top 0.203: N8.P$2 107.58,37.46 v107.78,37.5
  Bottom 0.203: v107.78,37.5 108.89,37.5 R48.1 108.93,37.51 110.09,38.67 110.09,40.62 108.88,41.84 108.88,43.14 111.56,45.83 117.08,45.83 117.97,46.72 117.97,59.07 117.16,59.88 IN_4.6
IN_1  (via drill 0.3)
  Top 0.203: v22.67,10.85 22.67,13.49 23.64,14.46 25.19,14.46 29.25,18.52 v33.23,18.52 | v48.1,17.71 51.76,17.71 v55.05,21 | v62.48,26.73 62.48,32.62 v65.49,35.63
  Bottom 0.203: IN_1.7 17.88,10.03 18.65,10.81 22.63,10.81 v22.67,10.85 | 33.76,18.52 36.64,21.41 44.4,21.41 v48.1,17.71 | v55.05,21 56.75,21 v62.48,26.73 | v65.49,35.63 65.49,35.66 AVR.27 | v33.23,18.52 33.76,18.52 | 33.76,18.52 33.8,18.52
IN_2  (via drill 0.3)
  Top 0.203: v77.84,21.03 73.29,25.51 v72.52,26.28
  Bottom 0.203: IN_2.7 76.46,14.55 77.84,15.93 v77.84,21.03 | v72.52,26.28 72.52,27.5 AVR.28
IN_3  (via drill 0.3)
  Top 0.203: v108.31,22.99 90.47,22.99 v90.11,23.36 | v79.67,28.27 v70.57,37.38 | v58.74,41.36 61.67,44.28 64.67,44.28 67.64,41.32 v67.64,40.38
  Bottom 0.203: IN_3.7 112.69,24.01 111.03,22.34 108.96,22.34 v108.31,22.99 | v90.11,23.36 84.58,23.36 v79.67,28.27 | v70.57,37.38 70.57,37.46 v67.64,40.38 | v58.74,41.36 57.53,41.36 AVR.12
IN_4  (via drill 0.3)
  Top 0.203: v114.6,58.42 114.6,62.52 v112.45,64.67 | v71.42,57.93 67.56,57.93 v54.88,45.26 | v110.99,66.06 89.78,66.06 v89.74,66.1
  Bottom 0.203: IN_4.7 113.79,59.23 v114.6,58.42 | v54.88,45.26 54.88,45.13 AVR.13 | v112.45,64.67 112.37,64.67 v110.99,66.06
  Bottom 0.254: v71.42,57.93 73.41,57.93 79.58,64.11 87.75,64.11 v89.74,66.1
IN_LOAD  (via drill 0.3)
  Top 0.203: v70.65,32.05 v70.65,21.53 62.6,13.49 v62.6,13.32 | v82.27,23.32 85.03,26.08 v106.6,26.08 108.22,27.71 v116.67,27.71 | v26.49,8.73 v31.73,8.73 | v45.62,8.69 v53.14,8.69 | v117.72,63.12 119.86,63.12 v121.02,61.95 | v119.72,47.65 119.72,41.19 v120.33,40.58
  Bottom 0.203: IN_2.1 v70.65,21.53 | v70.65,21.53 | v70.65,32.05 70.65,32.76 AVR.25 | IN_3.1 107.21,25.47 v106.6,26.08 | v82.27,23.32 72.43,23.32 v70.65,21.53 | IN_1.1 v26.48,8.74 v26.49,8.73 | v31.73,8.73 45.58,8.73 v45.62,8.69 | v53.14,8.69 57.97,8.69 v62.6,13.32 | v121.02,61.95 121.02,48.95 v119.72,47.65 | v120.33,40.58 120.33,31.36 v116.67,27.71 | IN_4.1 117.63,63.13 117.7,63.2 v117.72,63.12
IO_CLK  (via drill 0.3)
  Top 0.203: v109.44,23.73 109.44,18.93 v110.26,18.12 | v21.12,6.74 20.39,7.47 v20.39,12.43 21.08,13.12 21.08,16.21 v21.04,16.25 | v93.07,51.63 v93.07,49.03 | v66.5,21.21 66.5,36.2 v63.25,39.45 | v94.94,62.48 94.9,62.48 91.28,58.87 91.28,53.75 v90.47,52.93 | v30.18,31.97 30.18,29.45 21.04,20.31 v21.04,18.2 | v52.16,40.91 53.5,40.91 v61.22,48.63 | v94.66,27.5 88.6,27.5 v87.1,29.01 | v82.83,43.59 82.83,44 80.44,46.39 73.86,46.39 v73.12,45.66 | v77.9,50.95 81.5,50.95 v81.55,51
  Bottom 0.203: IN_4.2 IN_4.15 v94.94,62.48 | v109.44,23.73 IN_3.2 109.44,26.65 108.63,27.46 94.7,27.46 v94.66,27.5 | v110.26,18.12 109.44,18.93 IN_3.15 | IN_2.2 70.61,17.8 70.61,17.79 IN_2.15 66.54,17.8 66.54,21.17 v66.5,21.21 | IN_1.15 21.12,13.16 v20.39,12.43 | v21.12,6.74 IN_1.2 | 68.25,44.48 64.66,40.89 AVR.23 63.25,39.46 v63.25,39.45 | 68.25,44.48 72.76,44.48 | 72.76,44.48 74.99,44.48 75.72,45.22 SR_OUT3.11 75.72,48.79 77.35,50.42 77.37,50.42 v77.9,50.95 | 89.33,50.41 89.38,50.45 | 89.38,50.45 91.16,52.16 | 91.16,52.16 92.54,52.16 v93.07,51.63 | v93.07,49.03 95.71,49.03 96.44,48.3 SR_OUT2.11 | SR_OUT2.11 96.48,47.08 | SR_OUT2.11 | v90.47,52.93 91.16,52.16 | SR_OUT1.11 38.27,40.06 | 38.27,40.06 v30.18,31.97 | 38.27,40.06 51.31,40.06 v52.16,40.91 | v61.22,48.63 64.11,48.63 68.25,44.48 | v87.1,29.01 87.1,40.75 84.78,43.06 83.36,43.06 v82.83,43.59 | v73.12,45.66 72.76,45.26 72.76,44.48 | v81.55,51 87.7,51 88.3,50.4 89.32,50.4 89.38,50.45 | v21.04,16.25 v21.04,18.2
MISO3
  Bottom 0.203: CONNECTOR.79 85.09,77.74 83.95,76.6
  Bottom 0.254: SJ1.1 78.35,71 83.95,76.6
MISO_AVR
  Bottom 0.203: PROGRAMMING_CONNECTOR.9
  Bottom 0.254: 65.35,59.98 ADUM.11 | AVR.16 59.15,44.28 57.77,45.66 57.77,54.03 59.64,55.9 61.51,55.9 63.46,57.85 64.92,57.85 65.33,58.26 65.33,59.71 ADUM.11 | PROGRAMMING_CONNECTOR.9 14.5,81.7 16.29,79.78 16.3,79.52 16.3,74.9 18.3,72.9 21.61,69.59 36.39,69.59 39.4,72.6 52.74,72.6 58.34,67 61.36,63.98 63.91,63.98 65.33,62.56 65.33,59.73 ADUM.11
MOSI3  (via drill 0.3)
  Top 0.254: v78.39,72.3 v82.91,72.3
  Bottom 0.203: CONNECTOR.81 86.36,77.76 84.65,76.05
  Bottom 0.254: SJ2.1 v78.39,72.3 | v82.91,72.3 82.91,74.31 84.65,76.05
MOSI_AVR  (via drill 0.3)
  Top 0.254: PROGRAMMING_CONNECTOR.1 v16.1,73
  Bottom 0.254: AVR.15 58.59,43.71 57.24,45.05 57.24,54.32 59.39,56.47 61.1,56.47 62.81,58.17 ADUM.13 62.81,59.95 62.81,61.83 61.66,62.98 60.79,62.98 57.85,66 57.83,66 52.18,71.57 40.31,71.57 40.25,71.55 | 40.25,71.55 40.04,71.45 36.92,68.33 20.76,68.33 17.3,71.79 17.3,71.8 v16.1,73 | 40.26,71.55 40.25,71.55
N$1  (via drill 0.3)
  Top 0.203: A5.P$2 106.29,5.46 v106.92,6.09
  Bottom 0.203: v106.92,6.09 106.89,6.09 R35.1 112.01,12.98 IN_3.11
N$2  (via drill 0.3)
  Top 0.203: A3.P$2 103.56,12.46 v103.19,12.84
  Bottom 0.203: v103.19,12.84 104.33,13.97 104.29,13.97 | 104.29,13.97 104.24,13.97 | IN_3.12 111.36,17.11 110.5,16.25 106.57,16.25 R36.1 104.29,13.97
N$3
  Bottom 0.203: SR_OUT1.6 38.27,54.2 LCD.14
N$4
  Bottom 0.203: SR_OUT1.5 37.62,54.52 38.59,55.49 38.59,56.94 LCD.13
N$5
  Bottom 0.305: TRIMPOT.2 13.8,54.77 13.08,55.49 13.08,56.95 LCD.3
N$6
  Bottom 0.203: SR_OUT1.7 38.92,52.98 39.49,53.54 40.62,53.54 41.11,53.06 41.11,52.16 41.15,52.12 | 41.15,52.12 41.19,52.08 43.04,52.08 LCD_BACKLIGHT_FET.1 | R49.2 41.14,52.11 41.15,52.12
N$7
  Bottom 0.203: LCD_BACKLIGHT_FET.3 R50.2
N$8
  Bottom 0.203: R50.1 45.73,56.58 LCD.16
  Bottom 0.305: 46.11,56.96 LCD.16
N$9
  Bottom 0.203: SR_OUT1.4 36.97,56.02 LCD.12
N$10
  Bottom 0.203: SR_OUT1.3 36.32,54.13 LCD.11
N$11
  Bottom 0.203: SR_OUT1.2 35.67,52.89 33.72,54.84 22.91,54.84 LCD.6
N$12
  Bottom 0.508: D1.A 117.05,65.95 117.7,65.3 120.81,65.3 POWER_CONNECTOR.P$2
N$13
  Bottom 0.203: SR_OUT1.1 35.02,52.57 33.39,54.19 18.48,54.19 LCD.4
N$14
  Bottom 0.381: C1.+ 108.49,69.71 | D2.C
  Bottom 0.508: VOLTAGE_REGULATOR.1 D1.C 115.41,71.81 114.8,71.2 C3.1 114.73,66.8 113.6,66.8 112.59,67.81 D2.C
  Bottom 0.584: 108.49,69.71 110.4,67.8 D2.C
N$17  (via drill 0.3)
  Top 0.203: E1.B 30.81,4 37.7,10.89 37.74,10.89 49.97,23.12 49.97,23.28 v49.4,23.85 | v59.43,24.9 v59.39,30.75
  Bottom 0.203: v49.4,23.85 51.07,23.85 53.14,21.77 56.83,21.73 59.43,24.33 v59.43,24.9 | v59.39,30.75 59.39,32.36 AVR.32
N$20
  Bottom 0.254: C4.2 49.48,33.39 49.48,33.43 | 49.48,33.43 48.47,34.45 | 48.47,34.49 48.47,34.45 | 49.48,33.43 50.44,33.43 AVR.8 | Y1.1 48.47,34.45
N$21  (via drill 0.3)
  Top 0.254: v79.69,73.64 v88.43,73.64
  Bottom 0.203: v88.43,73.64 89.15,73.64 92.27,76.75 93.31,76.75 94.44,77.89 94.44,79.32 93.7,80.07 87.3,80.07 86.35,79.13 86.36,79.12 CONNECTOR.82
  Bottom 0.254: SJ3.1 v79.69,73.64
N$22  (via drill 0.3)
  Top 0.203: v81.06,74.9 85.64,74.9 v85.67,74.94
  Bottom 0.203: SJ4.1 v81.06,74.9 | CONNECTOR.80 85.09,79.2 86.48,80.59 100.17,80.59 102.83,77.92 102.83,72.86 100.78,70.81 88.72,70.81 85.67,73.89 v85.67,74.94
N$23
  Bottom 0.254: C2.2 54.4,28.52 | Y1.2 55.27,27.6 55.25,27.62 55.25,27.67 54.4,28.52 | 54.4,28.52 54.36,28.52 51.15,31.73 51.15,32.34 52.12,33.31 52.12,33.99 AVR.7
N$24  (via drill 0.3)
  Top 0.203: E1.A 19,4.05 20.39,5.44 31.44,5.44 47.82,21.82 47.82,27.95 v49.36,29.49 | v51.8,29.49 v54.07,31.77
  Bottom 0.203: v49.36,29.49 v51.8,29.49 | v54.07,31.77 54.62,31.22 54.68,31.22 54.75,31.15 56.5,31.15 58.6,33.25 58.7,33.75 59.15,34.2 59.12,34.2 | 59.1,34.2 59.12,34.2 | 59.12,34.2 AVR.1
N$25  (via drill 0.3)
  Top 0.203: E2.B 42.5,14.22 51.02,22.75 51.02,27.22 v55.63,31.82
  Bottom 0.203: v55.63,31.82 55.98,32.19 56.29,32.19 57.95,33.9 58,34.21 AVR.2
N$27  (via drill 0.3)
  Top 0.203: E2.A 37.5,9.92 50.54,22.95 50.54,35.55 v52.89,37.9
  Bottom 0.203: v52.89,37.9 52.89,38 AVR.9
N$28  (via drill 0.3)
  Top 0.203: v125.7,63.1 125.7,61.9
  Top 0.508: LED1.C 125.7,61.9
  Bottom 0.203: R52.2 124,61.9
  Bottom 0.254: 124,61.9 124,62.8 124.3,63.1 v125.7,63.1
N$29  (via drill 0.3)
  Top 0.254: v65.16,72.3 63.15,72.3 v62.79,71.94
  Bottom 0.254: SJ2.2 v65.16,72.3 | v62.79,71.94 62.79,69.15 62.82,69.12 ADUM.4 | ADUM.4 | ADUM.4
N$30  (via drill 0.3)
  Top 0.203: E3.A 56,15.86 57.93,17.79 57.93,37.66 v56.71,38.88
  Bottom 0.203: v56.71,38.88 56.71,39.91 AVR.10
N$31
  Bottom 0.254: SJ1.2 65.62,71 65.36,70.74 65.36,69.14 ADUM.6
N$32  (via drill 0.3)
  Top 0.203: E3.B 61,15.25 58.46,17.79 58.46,38.15 59.23,38.92 59.23,39.41 v58.58,40.06
  Bottom 0.203: v58.58,40.06 57.7,40.06 AVR.11
N$33
  Bottom 0.203: SR_OUT2.15 99.05,43.79 100.34,42.49 100.34,35.1 95.79,30.55 93.97,30.55 R7.1
N$34
  Bottom 0.203: SR_OUT2.1 99.7,36 95.79,32.09 R8.1
N$35
  Bottom 0.203: SR_OUT2.2 99.05,36.89 95.79,33.64 93.97,33.64 R9.1
N$36
  Bottom 0.203: SR_OUT2.3 98.4,37.71 95.79,35.1 R10.1
N$37
  Bottom 0.203: SR_OUT2.4 97.75,38.52 95.79,36.56 93.96,36.56 R11.1
N$38
  Bottom 0.203: SR_OUT2.5 97.1,39.41 95.79,38.11 93.94,38.11 R12.1
N$39
  Bottom 0.203: SR_OUT2.6 96.45,40.23 96.44,40.22 96.44,39.37 95.75,38.67 94.94,38.67 94.25,39.37 93.95,39.37 R13.1
N$40  (via drill 0.3)
  Top 0.203: v97.09,43.96 v97.09,48.59
  Bottom 0.203: SR_OUT2.7 95.8,43.96 v97.09,43.96 | R14.1 93.92,42.25 92.87,43.31 91,43.31 89.29,45.01 89.29,47.61 91.45,49.77 96.28,49.77 97.09,48.95 v97.09,48.59
N$41  (via drill 0.3)
  Top 0.406: LED17.A v91.2,30.59
  Bottom 0.406: v91.2,30.59 R7.2
N$42  (via drill 0.3)
  Top 0.406: LED18.A v91.2,32.09
  Bottom 0.406: v91.2,32.09 R8.2
N$43  (via drill 0.3)
  Top 0.406: LED19.A v91.2,33.59
  Bottom 0.406: v91.2,33.59 R9.2
N$44  (via drill 0.3)
  Top 0.406: LED20.A v91.2,35.09
  Bottom 0.406: v91.2,35.09 R10.2
N$45  (via drill 0.3)
  Top 0.406: LED21.A v91.2,36.59
  Bottom 0.406: v91.2,36.59 R11.2
N$46  (via drill 0.3)
  Top 0.406: LED22.A v91.2,38.09
  Bottom 0.406: v91.2,38.09 R12.2
N$47  (via drill 0.3)
  Top 0.406: LED23.A v91.2,39.59
  Bottom 0.203: 92.2,39.59 92.22,39.57 92.22,39.59 R13.2
  Bottom 0.406: v91.2,39.59 92.2,39.59
N$48  (via drill 0.3)
  Top 0.406: LED24.A v91.2,41.09
  Bottom 0.406: v91.2,41.09 R14.2
N$49
  Bottom 0.203: SR_OUT3.15 78.33,44.04 80.28,42.09 80.28,41.14 R17.1
N$50
  Bottom 0.203: SR_OUT3.1 78.97,40.06 79.46,39.57 80.25,39.57 | 80.28,39.57 80.25,39.57 | 80.25,39.57 R18.1
N$51
  Bottom 0.203: SR_OUT3.2 78.33,39.24 79.46,38.11 80.21,38.11 R19.1
N$52
  Bottom 0.203: SR_OUT3.3 77.67,38.35 79.46,36.56 80.19,36.56 R20.1
N$53
  Bottom 0.203: SR_OUT3.4 77.03,37.54 79.46,35.1 80.22,35.1 R21.1
N$54
  Bottom 0.203: SR_OUT3.5 76.38,36.64 79.46,33.56 80.19,33.56 R22.1
N$55
  Bottom 0.203: SR_OUT3.6 75.72,35.83 79.46,32.09 R23.1
N$56
  Bottom 0.203: SR_OUT3.7 75.08,35.02 79.46,30.63 80.19,30.63 R24.1
N$57  (via drill 0.3)
  Top 0.406: v82.95,41.09 LED25.A 84.08,41.09
  Bottom 0.406: R17.2 v82.95,41.09
N$58  (via drill 0.3)
  Top 0.406: LED26.A v82.95,39.59
  Bottom 0.406: v82.95,39.59 R18.2
N$59  (via drill 0.3)
  Top 0.406: v82.95,38.09 LED27.A
  Bottom 0.406: R19.2 v82.95,38.09
N$60  (via drill 0.3)
  Top 0.406: v82.95,36.59 LED28.A
  Bottom 0.406: R20.2 v82.95,36.59
N$61  (via drill 0.3)
  Top 0.406: v82.95,35.09 LED29.A
  Bottom 0.406: R21.2 v82.95,35.09
N$62  (via drill 0.3)
  Top 0.406: v82.95,33.59 LED30.A
  Bottom 0.406: R22.2 v82.95,33.59
N$63  (via drill 0.3)
  Top 0.406: v82.95,32.09 LED31.A
  Bottom 0.406: R23.2 v82.95,32.09
N$64  (via drill 0.3)
  Top 0.406: v82.95,30.59 LED32.A
  Bottom 0.406: R24.2 v82.95,30.59
N$65  (via drill 0.3)
  Top 0.254: v34.73,64.92 45.7,64.92 v51.84,58.78 | v57.85,57.73 61.42,57.73 v63.62,55.53 | v68.7,49.93 68.7,48.95 65.61,45.87 65.61,44.28 69.55,40.34 69.55,39.65 68.13,38.23 66.95,38.23 63.74,41.44 61.83,41.44 v61.18,40.79
  Bottom 0.254: v34.73,64.92 34.66,65 34.65,65 | v51.84,58.78 56.79,58.78 v57.85,57.73 | v63.62,55.53 63.62,55.01 v68.7,49.93 | v61.18,40.79 61.18,39.37 62.2,38.35 62.2,36.69 AVR.29 | D3.A 17.6,68 20.6,65 34.65,65 | 34.65,65 v34.73,64.92
  Bottom 0.406: D3.A 15.5,66 15.5,65.5 D4.A 12.35,65.65 R51.1
N$67  (via drill 0.3)
  Top 0.254: RESET.P$4 17.76,67.06 17.5,66.8 v17.5,65.9
  Top 1.42: RESET.P$3 RESET.P$4
  Bottom 0.254: v17.5,65.9 D3.C
N$266  (via drill 3.65 pad 7.8)  (1 unrouted)
  other vias: 28.62,75.15 98.35,75.15
OUT
  Bottom 0.203: AVR.26 64.66,37.64 63.86,38.43 63.86,38.76 64.31,39.2 65.28,39.2 69.43,43.35 75.6,43.35 77.67,45.42 SR_OUT3.14
OUT_DAISY  (via drill 0.3)
  Top 0.203: v91.04,50.33 90.35,49.68 v87.3,49.68 | v99.65,49.64 99.65,51.47 v99.61,51.59 | v75.52,49.68 v82.14,49.68
  Bottom 0.203: SR_OUT3.9 74.42,48.59 v75.52,49.68 | 98.39,47.04 SR_OUT2.14 | SR_OUT2.14 | SR_OUT2.14 98.39,48.38 v99.65,49.64 | v99.61,51.59 98.47,51.59 97.22,50.33 v91.04,50.33 | v82.14,49.68 v87.3,49.68
OUT_DAISY2  (via drill 0.3)
  Top 0.203: v90.96,48.22 v82.14,48.22 | v61.3,53.3 55.09,53.3 v50.7,48.91 | v41.97,42.82 37.01,42.82 v36.32,43.51 | v69.35,46.23 71.47,46.23 73.7,44 80.64,44 v80.68,43.96
  Bottom 0.203: SR_OUT2.9 93.61,47.08 92.46,48.22 v90.96,48.22 | v82.14,48.22 82.14,45.42 v80.68,43.96 | v69.35,46.23 68.37,46.23 v61.3,53.3 | v50.7,48.91 48.06,48.91 v41.97,42.82 | v36.32,43.51 SR_OUT1.14
OUT_LATCH  (via drill 0.3)
  Top 0.203: v90.35,47.25 v87.18,47.25 | v84.34,47.25 78.57,47.25 v76.94,48.91 75.2,47.17 v71.74,47.17 | v36.77,41.48 47.65,41.48 v49.24,43.06 | v55.86,49.48 57.81,49.48 v60.37,52.04
  Bottom 0.203: AVR.24 65.22,40.32 68.82,43.92 75.08,43.92 76.38,45.22 SR_OUT3.12 76.38,46.96 | SR_OUT2.12 97.1,45.26 96.4,44.57 94.17,44.57 93.15,45.58 93.15,46.48 92.38,47.25 v90.35,47.25 | v87.18,47.25 v84.34,47.25 | v76.94,48.91 76.94,48.95 76.38,48.34 76.38,46.96 | 76.38,46.96 76.33,46.92 | SR_OUT1.12 37.62,42.33 v36.77,41.48 | v49.24,43.06 49.44,43.06 v55.86,49.48 | v60.37,52.04 61.59,52.04 68.17,45.46 70.04,45.46 v71.74,47.17
RESET
  Bottom 0.406: D4.C 14,70.5 15,71.5 15,76.13 PROGRAMMING_CONNECTOR.5
RX  (via drill 0.3)
  Top 0.203: PROGRAMMING_CONNECTOR.10 7.64,80.28 7.07,79.75 6.5,79.26 6.5,60.86 4.47,58.83 4.47,56.63 6.5,54.6 6.5,50.66 v6.66,50.5 | v13.41,42.09 31.16,42.09 v36.77,36.48 | v43.55,36.77 50.21,36.77 v50.94,37.5 | v52.41,36.44 54.27,36.44 56.72,33.99 57.12,33.59 v57.12,29.98 | v60.41,29.66 61.55,30.79 61.55,32.42 61.02,32.95 v61.02,36.73
  Bottom 0.203: v6.66,50.5 6.66,48.83 v13.41,42.09 | v36.77,36.48 43.27,36.48 v43.55,36.77 | v50.94,37.5 51.35,37.5 v52.41,36.44 | v57.12,29.98 57.44,29.66 v60.41,29.66 | v61.02,36.73 62.36,35.38 | 62.44,35.3 62.4,35.34 | AVR.30 62.36,35.38 | 62.36,35.38 62.36,35.47 62.4,35.42 62.4,35.34 | 62.4,35.34 AVR.30 | AVR.30
SCK_AVR  (via drill 0.3)
  Top 0.254: v64.11,56.96 v64.11,62.73
  Bottom 0.203: PROGRAMMING_CONNECTOR.7 13.08,80.62
  Bottom 0.254: AVR.17 61.24,44.26 58.3,47.21 58.3,53.58 59.96,55.25 61.67,55.25 63.38,56.96 v64.11,56.96 | 64.07,59.88 64.05,59.9 ADUM.12 64.03,59.76 64.03,61.83 63.62,62.24 | 13.08,80.62 15.7,78 15.7,74.5 17.9,72.3 17.9,72.29 21.25,68.94 36.62,68.94 38.21,70.53 39.9,72.1 52.46,72.1 61.07,63.49 62.36,63.49 63.62,62.24 | v64.11,62.73 63.62,62.24
SS3
  Bottom 0.254: SJ4.2 64.35,74.9 61.52,72.08 ADUM.3 | ADUM.3 | ADUM.3
SS_AVR
  Bottom 0.254: AVR.14 56.67,44.48 56.67,54.72 58.99,57.04 60.45,57.04 61.51,58.09 61.51,59.7 ADUM.14
TX  (via drill 0.3)
  Top 0.203: PROGRAMMING_CONNECTOR.8 10.42,80.62 7.03,77.23 7.03,60.12 v5.4,58.5 | v12.59,40.95 31.04,40.95 40.67,31.32 41.44,31.32 v46.56,26.2 | v60.12,26.77 60.77,26.77 v61.63,27.62
  Bottom 0.203: v5.4,58.5 5.4,48.14 v12.59,40.95 | AVR.31 61.85,34.79 62.89,33.76 62.89,30.39 61.63,29.13 v61.63,27.62 | v46.56,26.2 49.44,26.2 53.46,22.18 56.67,22.18 58.58,24.09 58.58,25.23 v60.12,26.77
(copper drawn outside any net)
  shapes: Bottom area x1, Bottom circle x15, Top area x1, Top circle x4

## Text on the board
Top: RX | MISO | TX | SCK | GND | RESET | GND | GND | 5V | MOSI | 7 | 8 | 9 | 4 | 5 | 6 | 1 | 2 | 3 | + | - | 0 | . | C | D | A | B
Bottom: SS | SCK | MOSI | MISO | Controller | DSP | REV B | Tibor | Simon | 2013
tStop: 7 | 8 | 9 | 4 | 5 | 6 | 1 | 2 | 3 | + | - | 0 | . | C | D | A | B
